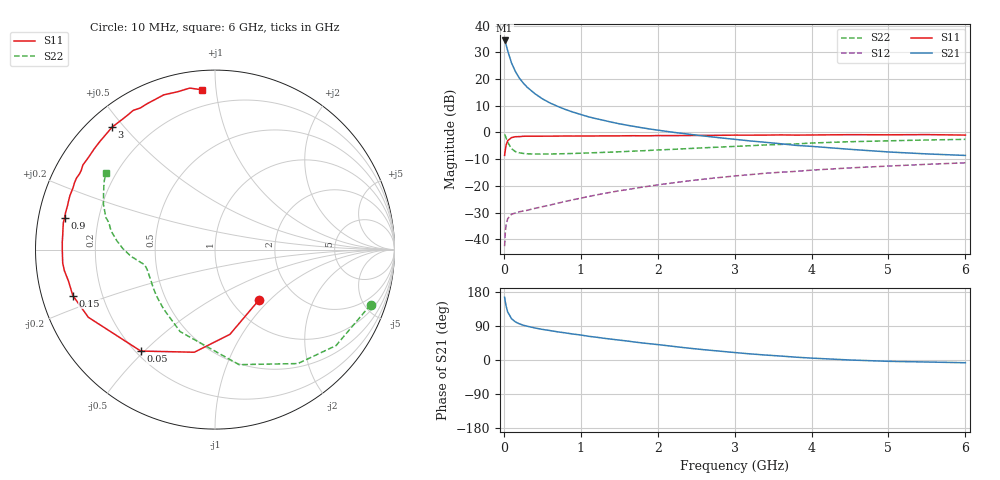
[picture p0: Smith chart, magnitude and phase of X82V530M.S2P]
! SIEMENS Small Signal Semiconductors
! BFP136W
! Si NPN RF Bipolar Junction Transistor in SOT343
! VCE = 2.5 V  IC = 30 mA
! Common Emitter S-Parameters:  September  1994
# GHz  S  MA  R  50
!  f  S11  S21  S12  S22
! GHz  MAG  ANG  MAG  ANG  MAG  ANG  MAG  ANG
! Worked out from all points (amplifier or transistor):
!   40 points, 10 MHz to 6 GHz, reference 50 ohm
!   highest |S21| = 34.5 dB at 10 MHz (marker M1)
!   |S21| within 3 dB of that: start of sweep to 42.07 MHz
!   unconditionally stable (mu >= 1): 752.5 MHz to 2.804 GHz
!   at 200 MHz: K = 0.43, MSG = 25.1 dB, |S12| = -29.7 dB
!   at 1.5 GHz: K = 1.14, MAG = 10.3 dB, |S12| = -21.9 dB
!   at 6 GHz: K = 0.98, MSG = 1.4 dB, |S12| = -11.4 dB
!   S11 on the Smith chart (normalised r, x): 10 MHz: 1.34, -0.86; 50 MHz: 0.22, -0.49; 150 MHz: 0.09, -0.16; 900 MHz: 0.08, +0.10; 3 GHz: 0.07, +0.46; 6 GHz: 0.10, +0.92
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0.01  0.3722 -48.5  52.94 165.6  0.0074 74.6  0.9198 -19.5
0.02  0.4794 -80.0  48.34 152.5  0.014 64.9  0.8607 -38.4
0.03  0.5833 -101.4  43.68 141.9  0.0187 55.5  0.7849 -54.0
0.05  0.7005 -126.2  33.89 126.8  0.0242 41.7  0.6547 -78.2
0.1  0.8003 -151.9  20.07 108.9  0.0293 30.2  0.4964 -113.1
0.15  0.8324 -162.1  13.89 100.6  0.031 28.2  0.4379 -130.8
0.2  0.8352 -168.0  10.51 95.6  0.0326 28.0  0.4163 -141.3
0.25  0.8476 -172.1  8.503 92.0  0.0337 29.0  0.4052 -148.0
0.3  0.8518 -175.0  7.118 89.3  0.0347 30.5  0.3981 -152.6
0.4  0.8507 -179.5  5.368 84.7  0.0377 34.3  0.3941 -158.5
0.5  0.852 177.2  4.28 80.8  0.0406 38.0  0.3933 -162.2
0.6  0.8522 174.7  3.57 77.7  0.0436 40.6  0.3952 -164.4
0.7  0.855 172.0  3.078 74.3  0.0472 43.9  0.3972 -165.8
0.9  0.8567 168.0  2.404 68.5  0.0548 47.6  0.4036 -168.2
1.1  0.8572 163.4  1.964 62.6  0.0629 50.6  0.4132 -169.4
1.5  0.8626 156.6  1.455 52.5  0.0807 53.8  0.4344 -171.9
2.2  0.8722 144.0  1.008 36.0  0.1136 53.2  0.4826 -177.1
3  0.8911 130.1  0.744 19.7  0.1529 48.3  0.5482 175.0
3.2  0.8903 126.8  0.694 16.2  0.162 46.6  0.5644 172.7
4.5  0.9083 108.3  0.483 0.0  0.2167 35.1  0.6709 157.9
5.5  0.9108 98.9  0.396 -5.3  0.2529 26.9  0.723 148.8
6  0.8929 94.5  0.371 -7.2  0.2701 22.4  0.7421 145.0
